| IBIS file stm32l0_71_72_73_81_82_83_lqfp48.ibs
| Created by s2ibis version 1.1 (customized version)
| North Carolina State University, ERL, 2006
[IBIS ver] 4.2
[File name] stm32l0_71_72_73_81_82_83_lqfp48.ibs
[File Rev] 1.0
[Date]  14-03-2016
[Source] Data Created at STMicroelectronics
[Notes]  File originated from ELDO simulations.
[Disclaimer]  This information is for modeling purpose only and is
   not guaranted. The information is subject to change without
   notice.
[Copyright] Copyright 2016 STMicroelectronics Inc.
|   Component stm32l0_71_72_73_81_82_83_lqfp48
[Component] stm32l0_71_72_73_81_82_83_lqfp48
[Manufacturer] STMicroelectronics
[Package]
| variable   typ   min   max
R_pkg   0.0   0.0   0.0
L_pkg   0.0H   0.0H   0.0H
C_pkg   0.0F   0.0F   0.0F
[Pin]  signal_name   model_name   R_pin   L_pin   C_pin
1 VLCD POWER   0.053   3.42534E-09   90.4E-15
2 PC13 io8p_wsudq_ls_ft_v33   48.4E-3   2.9E-9   64.4E-15
3 PC14-OSC32_IN io8p_wsudq_ls_ft_v33   44.7E-3   2.5E-9   43.7E-15
4 PC15-OSC32_OUT io8p_sudq_ls_tc_esdft 41.9E-3   2.2E-9   28.1E-15
5 PH0-OSC_IN io8p_sudq_ls_tc_esdft   40.1E-3   2.0E-9   17.7E-15
6 PH1-OSC_OUT io8p_sudq_ls_tc_esdft   0.03913   1.89021E-09   12.5E-15
7 NRST ioreset_ft_v33   0.03913   1.89021E-09   12.5E-15
8 VSSA GND   40.1E-3   2.0E-9   17.8E-15
9 VDDA POWER   41.9E-3   2.2E-9   28.2E-15
10 PA0 io8p_wsudq_ls_ft_v33   44.7E-3   2.5E-9   43.8E-15
11 PA1 io8p_wsudq_lcd4_ls_ft  48.4E-3   2.9E-9   64.6E-15
12 PA2 io8p_wsudq_lcd4_ls_ft  0.053   3.42534E-09   90.4E-15
13 PA3 io8p_wsudq_lcd4_ls_ft  0.053   3.4E-9   90.4E-15
14 PA4 io8p_wsudq_i2cin_ls_ft 48.4E-3   2.9E-9   64.4E-15
15 PA5 io8p_wsudq_i2cin_ls_ft 44.7E-3   2.5E-9   43.7E-15
16 PA6 io8p_wsudq_lcd4_ls_ft  41.9E-3   2.2E-9   28.1E-15
17 PA7 io8p_wsudq_lcd4_ls_ft  40.1E-3   2.0E-9   17.7E-15
18 PB0 io8p_wsudq_lcd4_ls_ft  0.03913   1.9E-9   12.5E-15
19 PB1 io8p_wsudq_lcd4_ls_ft  0.03913   1.9E-9   12.5E-15
20 PB2 io8p_wsudq_lcd4_ls_ft  40.1E-3   2.0E-9   17.8E-15
21 PB10 io8p_sudq_lcd4_i2cin_ls_ft   41.9E-3   2.2E-9   28.2E-15
22 PB11 io8p_sudq_lcd4_i2cin_ls_ft   44.7E-3   2.5E-9   43.8E-15
23 VSS GND   48.4E-3   2.9E-9   64.6E-15
24 VDD POWER   0.053   3.4E-9   90.4E-15
25 PB12 io8p_wsudq_lcd4_ls_ft   0.053   3.4E-9   90.4E-15
26 PB13 io8p_sudq_lcd4_i2cin_ls_ft   48.4E-3   2.9E-9   64.4E-15
27 PB14 io8p_sudq_lcd4_i2cin_ls_ft   44.7E-3   2.5E-9   43.7E-15
28 PB15 io8p_wsudq_lcd4_ls_ft   41.9E-3   2.2E-9   28.1E-15
29 PA8 io8p_sudq_lcd4_i2cin_ls_ft   40.1E-3   2.0E-9   17.7E-15
30 PA9 io8p_sudq_lcd4_i2cin_ls_ft   0.03913   1.9E-9   12.5E-15
31 PA10 io8p_sudq_lcd4_i2cin_ls_ft   0.03913   1.9E-9   12.5E-15
32 PA11 io8usb_ls_ft   40.1E-3   2.0E-9   17.8E-15
33 PA12 io8usb_ls_ft   41.9E-3   2.2E-9   28.2E-15
34 PA13 io8p_sudq_ls_ft   44.7E-3   2.5E-9   43.8E-15
35 VSS GND   48.4E-3   2.9E-9   64.6E-15
36 VDD_USB POWER   0.053   3.4E-9   90.4E-15
37 PA14 io8p_sudq_ls_ft   0.053   3.4E-9   90.4E-15
38 PA15 io8p_wsudq_lcd4_ls_ft   48.4E-3   2.9E-9   64.4E-15
39 PB3 io8p_wsudq_lcd4_ls_ft   44.7E-3   2.5E-9   43.7E-15
40 PB4 io8p_sudq_lcd4_i2cin_ls_ft 41.9E-3   2.2E-9   28.1E-15
41 PB5 io8p_wsudq_lcd4_ls_ft   40.1E-3   2.0E-9   17.7E-15
42 PB6 io8p_wsudq_i2cin_ls_ft   0.03913   1.9E-9   12.5E-15
43 PB7 io8p_wsudq_i2cin_ls_ft   0.03913   1.9E-9   12.5E-15
44 BOOT0 vpp_test_hv  40.1E-3   2.0E-9   17.8E-15
45 PB8 io8p_sudq_lcd4_i2cin_ls_ft   41.9E-3   2.2E-9   28.2E-15
46 PB9 io8p_sudq_lcd4_i2cin_ls_ft   44.7E-3   2.5E-9   43.8E-15
47 VSS GND   48.4E-3  2.9E-9   64.6E-15
48 VDD POWER   0.053   3.4E-9   90.4E-15
[Model Selector] io8p_sudq_ls_ft
io8p00_sudq_ls_ft_pd_lv  "SPEED00 1P8V, PD=40kOhm"
io8p00_sudq_ls_ft_pu_lv  "SPEED00 1P8V, PU=40kOhm"
io8p00_sudq_ls_ft_lv  "SPEED00 1P8V"
io8p01_sudq_ls_ft_pd_lv  "SPEED01 1P8V, PD=40kOhm"
io8p01_sudq_ls_ft_pu_lv  "SPEED01 1P8V, PU=40kOhm"
io8p01_sudq_ls_ft_lv  "SPEED01 1P8V"
io8p10_sudq_ls_ft_pd_lv  "SPEED10 1P8V, PD=40kOhm"
io8p10_sudq_ls_ft_pu_lv  "SPEED10 1P8V, PU=40kOhm"
io8p10_sudq_ls_ft_lv  "SPEED10 1P8V"
io8p11_sudq_ls_ft_pd_lv  "SPEED11 1P8V, PD=40kOhm"
io8p11_sudq_ls_ft_pu_lv  "SPEED11 1P8V, PU=40kOhm"
io8p11_sudq_ls_ft_lv  "SPEED11 1P8V"
io8p00_sudq_ls_ft_pd  "SPEED00, PD=40kOhm"
io8p00_sudq_ls_ft_pu  "SPEED00, PU=40kOhm"
io8p00_sudq_ls_ft  "SPEED00"
io8p01_sudq_ls_ft_pd  "SPEED01, PD=40kOhm"
io8p01_sudq_ls_ft_pu  "SPEED01, PU=40kOhm"
io8p01_sudq_ls_ft  "SPEED01"
io8p10_sudq_ls_ft_pd  "SPEED10, PD=40kOhm"
io8p10_sudq_ls_ft_pu  "SPEED10, PU=40kOhm"
io8p10_sudq_ls_ft  "SPEED10"
io8p11_sudq_ls_ft_pd  "SPEED11, PD=40kOhm"
io8p11_sudq_ls_ft_pu  "SPEED11, PU=40kOhm"
io8p11_sudq_ls_ft  "SPEED11"
[Model Selector] io8p_sudq_ls_tc_esdft
io8p00_sudq_ls_tc_esdft_pd_lv  "SPEED00 1P8V, PD=40kOhm"
io8p00_sudq_ls_tc_esdft_pu_lv  "SPEED00 1P8V, PU=40kOhm"
io8p00_sudq_ls_tc_esdft_lv  "SPEED00 1P8V"
io8p01_sudq_ls_tc_esdft_pd_lv  "SPEED01 1P8V, PD=40kOhm"
io8p01_sudq_ls_tc_esdft_pu_lv  "SPEED01 1P8V, PU=40kOhm"
io8p01_sudq_ls_tc_esdft_lv  "SPEED01 1P8V"
io8p10_sudq_ls_tc_esdft_pd_lv  "SPEED10 1P8V, PD=40kOhm"
io8p10_sudq_ls_tc_esdft_pu_lv  "SPEED10 1P8V, PU=40kOhm"
io8p10_sudq_ls_tc_esdft_lv  "SPEED10 1P8V"
io8p11_sudq_ls_tc_esdft_pd_lv  "SPEED11 1P8V, PD=40kOhm"
io8p11_sudq_ls_tc_esdft_pu_lv  "SPEED11 1P8V, PU=40kOhm"
io8p11_sudq_ls_tc_esdft_lv  "SPEED11 1P8V"
io8p00_sudq_ls_tc_esdft_pd  "SPEED00, PD=40kOhm"
io8p00_sudq_ls_tc_esdft_pu  "SPEED00, PU=40kOhm"
io8p00_sudq_ls_tc_esdft  "SPEED00"
io8p01_sudq_ls_tc_esdft_pd  "SPEED01, PD=40kOhm"
io8p01_sudq_ls_tc_esdft_pu  "SPEED01, PU=40kOhm"
io8p01_sudq_ls_tc_esdft  "SPEED01"
io8p10_sudq_ls_tc_esdft_pd  "SPEED10, PD=40kOhm"
io8p10_sudq_ls_tc_esdft_pu  "SPEED10, PU=40kOhm"
io8p10_sudq_ls_tc_esdft  "SPEED10"
io8p11_sudq_ls_tc_esdft_pd  "SPEED11, PD=40kOhm"
io8p11_sudq_ls_tc_esdft_pu  "SPEED11, PU=40kOhm"
io8p11_sudq_ls_tc_esdft  "SPEED11"
[Model Selector] io8p_wsudq_i2cin_ls_ft
io8p00_wsudq_i2cin_ls_ft_pd_lv  "SPEED00 1P8V, PD=40kOhm"
io8p00_wsudq_i2cin_ls_ft_pu_lv  "SPEED00 1P8V, PU=40kOhm"
io8p00_wsudq_i2cin_ls_ft_lv  "SPEED00 1P8V"
io8p01_wsudq_i2cin_ls_ft_pd_lv  "SPEED01 1P8V, PD=40kOhm"
io8p01_wsudq_i2cin_ls_ft_pu_lv  "SPEED01 1P8V, PU=40kOhm"
io8p01_wsudq_i2cin_ls_ft_lv  "SPEED01 1P8V"
io8p10_wsudq_i2cin_ls_ft_pd_lv  "SPEED10 1P8V, PD=40kOhm"
io8p10_wsudq_i2cin_ls_ft_pu_lv  "SPEED10 1P8V, PU=40kOhm"
io8p10_wsudq_i2cin_ls_ft_lv  "SPEED10 1P8V"
io8p11_wsudq_i2cin_ls_ft_pd_lv  "SPEED11 1P8V, PD=40kOhm"
io8p11_wsudq_i2cin_ls_ft_pu_lv  "SPEED11 1P8V, PU=40kOhm"
io8p11_wsudq_i2cin_ls_ft_lv  "SPEED11 1P8V"
io8p00_wsudq_i2cin_ls_ft_pd  "SPEED00, PD=40kOhm"
io8p00_wsudq_i2cin_ls_ft_pu  "SPEED00, PU=40kOhm"
io8p00_wsudq_i2cin_ls_ft  "SPEED00"
io8p01_wsudq_i2cin_ls_ft_pd  "SPEED01, PD=40kOhm"
io8p01_wsudq_i2cin_ls_ft_pu  "SPEED01, PU=40kOhm"
io8p01_wsudq_i2cin_ls_ft  "SPEED01"
io8p10_wsudq_i2cin_ls_ft_pd  "SPEED10, PD=40kOhm"
io8p10_wsudq_i2cin_ls_ft_pu  "SPEED10, PU=40kOhm"
io8p10_wsudq_i2cin_ls_ft  "SPEED10"
io8p11_wsudq_i2cin_ls_ft_pd  "SPEED11, PD=40kOhm"
io8p11_wsudq_i2cin_ls_ft_pu  "SPEED11, PU=40kOhm"
io8p11_wsudq_i2cin_ls_ft  "SPEED11"
[Model Selector] io8p_wsudq_lcd4_ls_ft
io8p00_wsudq_lcd4_ls_ft_pd_lv  "SPEED00 1P8V, PD=40kOhm"
io8p00_wsudq_lcd4_ls_ft_pu_lv  "SPEED00 1P8V, PU=40kOhm"
io8p00_wsudq_lcd4_ls_ft_lv  "SPEED00 1P8V"
io8p01_wsudq_lcd4_ls_ft_pd_lv  "SPEED01 1P8V, PD=40kOhm"
io8p01_wsudq_lcd4_ls_ft_pu_lv  "SPEED01 1P8V, PU=40kOhm"
io8p01_wsudq_lcd4_ls_ft_lv  "SPEED01 1P8V"
io8p10_wsudq_lcd4_ls_ft_pd_lv  "SPEED10 1P8V, PD=40kOhm"
io8p10_wsudq_lcd4_ls_ft_pu_lv  "SPEED10 1P8V, PU=40kOhm"
io8p10_wsudq_lcd4_ls_ft_lv  "SPEED10 1P8V"
io8p11_wsudq_lcd4_ls_ft_pd_lv  "SPEED11 1P8V, PD=40kOhm"
io8p11_wsudq_lcd4_ls_ft_pu_lv  "SPEED11 1P8V, PU=40kOhm"
io8p11_wsudq_lcd4_ls_ft_lv  "SPEED11 1P8V"
io8p00_wsudq_lcd4_ls_ft_pd  "SPEED00, PD=40kOhm"
io8p00_wsudq_lcd4_ls_ft_pu  "SPEED00, PU=40kOhm"
io8p00_wsudq_lcd4_ls_ft  "SPEED00"
io8p01_wsudq_lcd4_ls_ft_pd  "SPEED01, PD=40kOhm"
io8p01_wsudq_lcd4_ls_ft_pu  "SPEED01, PU=40kOhm"
io8p01_wsudq_lcd4_ls_ft  "SPEED01"
io8p10_wsudq_lcd4_ls_ft_pd  "SPEED10, PD=40kOhm"
io8p10_wsudq_lcd4_ls_ft_pu  "SPEED10, PU=40kOhm"
io8p10_wsudq_lcd4_ls_ft  "SPEED10"
io8p11_wsudq_lcd4_ls_ft_pd  "SPEED11, PD=40kOhm"
io8p11_wsudq_lcd4_ls_ft_pu  "SPEED11, PU=40kOhm"
io8p11_wsudq_lcd4_ls_ft  "SPEED11"
[Model Selector] io8p_wsudq_ls_ft_v33
io8p00_wsudq_ls_ft_v33_pd_lv  "SPEED00 1P8V, PD=40kOhm"
io8p00_wsudq_ls_ft_v33_pu_lv  "SPEED00 1P8V, PU=40kOhm"
io8p00_wsudq_ls_ft_v33_lv  "SPEED00 1P8V"
io8p01_wsudq_ls_ft_v33_pd_lv  "SPEED01 1P8V, PD=40kOhm"
io8p01_wsudq_ls_ft_v33_pu_lv  "SPEED01 1P8V, PU=40kOhm"
io8p01_wsudq_ls_ft_v33_lv  "SPEED01 1P8V"
io8p10_wsudq_ls_ft_v33_pd_lv  "SPEED10 1P8V, PD=40kOhm"
io8p10_wsudq_ls_ft_v33_pu_lv  "SPEED10 1P8V, PU=40kOhm"
io8p10_wsudq_ls_ft_v33_lv  "SPEED10 1P8V"
io8p11_wsudq_ls_ft_v33_pd_lv  "SPEED11 1P8V, PD=40kOhm"
io8p11_wsudq_ls_ft_v33_pu_lv  "SPEED11 1P8V, PU=40kOhm"
io8p11_wsudq_ls_ft_v33_lv  "SPEED11 1P8V"
io8p00_wsudq_ls_ft_v33_pd  "SPEED00, PD=40kOhm"
io8p00_wsudq_ls_ft_v33_pu  "SPEED00, PU=40kOhm"
io8p00_wsudq_ls_ft_v33  "SPEED00"
io8p01_wsudq_ls_ft_v33_pd  "SPEED01, PD=40kOhm"
io8p01_wsudq_ls_ft_v33_pu  "SPEED01, PU=40kOhm"
io8p01_wsudq_ls_ft_v33  "SPEED01"
io8p10_wsudq_ls_ft_v33_pd  "SPEED10, PD=40kOhm"
io8p10_wsudq_ls_ft_v33_pu  "SPEED10, PU=40kOhm"
io8p10_wsudq_ls_ft_v33  "SPEED10"
io8p11_wsudq_ls_ft_v33_pd  "SPEED11, PD=40kOhm"
io8p11_wsudq_ls_ft_v33_pu  "SPEED11, PU=40kOhm"
io8p11_wsudq_ls_ft_v33  "SPEED11"
[Model Selector] vpp_test_hv
vpp_test_hv_2p4  "Input Buffer 1P65V"
vpp_test_hv_3p3  "Input Buffer"
[Model Selector] io8usb_ls_ft
io8usb_ls_ft_dpdn_pu  "HS USB DP/DN IO + PU=1.2kOhm"
io8usb_ls_ft_dpdn  "HS USB DP/DN IO"
io8p00_ls_ft_pd_lv  "SPEED00 1P8V, PD=40kOhm"
io8p00_ls_ft_pu_lv  "SPEED00 1P8V, PU=40kOhm"
io8p00_ls_ft_lv  "SPEED00 1P8V"
io8p01_ls_ft_pd_lv  "SPEED01 1P8V, PD=40kOhm"
io8p01_ls_ft_pu_lv  "SPEED01 1P8V, PU=40kOhm"
io8p01_ls_ft_lv  "SPEED01 1P8V"
io8p10_ls_ft_pd_lv  "SPEED10 1P8V, PD=40kOhm"
io8p10_ls_ft_pu_lv  "SPEED10 1P8V, PU=40kOhm"
io8p10_ls_ft_lv  "SPEED10 1P8V"
io8p11_ls_ft_pd_lv  "SPEED11 1P8V, PD=40kOhm"
io8p11_ls_ft_pu_lv  "SPEED11 1P8V, PU=40kOhm"
io8p11_ls_ft_lv  "SPEED11 1P8V"
io8p00_ls_ft_pd  "SPEED00, PD=40kOhm"
io8p00_ls_ft_pu  "SPEED00, PU=40kOhm"
io8p00_ls_ft  "SPEED00"
io8p01_ls_ft_pd  "SPEED01, PD=40kOhm"
io8p01_ls_ft_pu  "SPEED01, PU=40kOhm"
io8p01_ls_ft  "SPEED01"
io8p10_ls_ft_pd  "SPEED10, PD=40kOhm"
io8p10_ls_ft_pu  "SPEED10, PU=40kOhm"
io8p10_ls_ft  "SPEED10"
io8p11_ls_ft_pd  "SPEED11, PD=40kOhm"
io8p11_ls_ft_pu  "SPEED11, PU=40kOhm"
io8p11_ls_ft  "SPEED11"
[Model Selector] io8p_sudq_lcd4_i2cin_ls_ft
io8p00_sudq_lcd4_i2cin_ls_ft_pd_lv  "SPEED00 1P8V, PD=40kOhm"
io8p00_sudq_lcd4_i2cin_ls_ft_pu_lv  "SPEED00 1P8V, PU=40kOhm"
io8p00_sudq_lcd4_i2cin_ls_ft_lv  "SPEED00 1P8V"
io8p01_sudq_lcd4_i2cin_ls_ft_pd_lv  "SPEED01 1P8V, PD=40kOhm"
io8p01_sudq_lcd4_i2cin_ls_ft_pu_lv  "SPEED01 1P8V, PU=40kOhm"
io8p01_sudq_lcd4_i2cin_ls_ft_lv  "SPEED01 1P8V"
io8p10_sudq_lcd4_i2cin_ls_ft_pd_lv  "SPEED10 1P8V, PD=40kOhm"
io8p10_sudq_lcd4_i2cin_ls_ft_pu_lv  "SPEED10 1P8V, PU=40kOhm"
io8p10_sudq_lcd4_i2cin_ls_ft_lv  "SPEED10 1P8V"
io8p11_sudq_lcd4_i2cin_ls_ft_pd_lv  "SPEED11 1P8V, PD=40kOhm"
io8p11_sudq_lcd4_i2cin_ls_ft_pu_lv  "SPEED11 1P8V, PU=40kOhm"
io8p11_sudq_lcd4_i2cin_ls_ft_lv  "SPEED11 1P8V"
io8p00_sudq_lcd4_i2cin_ls_ft_pd  "SPEED00, PD=40kOhm"
io8p00_sudq_lcd4_i2cin_ls_ft_pu  "SPEED00, PU=40kOhm"
io8p00_sudq_lcd4_i2cin_ls_ft  "SPEED00"
io8p01_sudq_lcd4_i2cin_ls_ft_pd  "SPEED01, PD=40kOhm"
io8p01_sudq_lcd4_i2cin_ls_ft_pu  "SPEED01, PU=40kOhm"
io8p01_sudq_lcd4_i2cin_ls_ft  "SPEED01"
io8p10_sudq_lcd4_i2cin_ls_ft_pd  "SPEED10, PD=40kOhm"
io8p10_sudq_lcd4_i2cin_ls_ft_pu  "SPEED10, PU=40kOhm"
io8p10_sudq_lcd4_i2cin_ls_ft  "SPEED10"
io8p11_sudq_lcd4_i2cin_ls_ft_pd  "SPEED11, PD=40kOhm"
io8p11_sudq_lcd4_i2cin_ls_ft_pu  "SPEED11, PU=40kOhm"
io8p11_sudq_lcd4_i2cin_ls_ft  "SPEED11"
[Model Selector] ioreset_ft_v33
ioreset_ft_v33_pu_lv  "ioreset 1P8V + PU=40kOhm"
ioreset_ft_v33_nopu_lv  "ioreset 1P8V"
ioreset_ft_v33_pu  "ioreset + PU=40kOhm"
ioreset_ft_v33_nopu  "ioreset"
| Models and submodels in the file (176): io8p00_sudq_ls_ft_pd_lv (I/O), io8p00_sudq_ls_ft_pu_lv (I/O), io8p00_sudq_ls_ft_lv (I/O), io8p01_sudq_ls_ft_pd_lv (I/O), io8p01_sudq_ls_ft_pu_lv (I/O), io8p01_sudq_ls_ft_lv (I/O), io8p10_sudq_ls_ft_pd_lv (I/O), io8p10_sudq_ls_ft_pu_lv (I/O), io8p10_sudq_ls_ft_lv (I/O), io8p11_sudq_ls_ft_pd_lv (I/O), io8p11_sudq_ls_ft_pu_lv (I/O), io8p11_sudq_ls_ft_lv (I/O), io8p00_sudq_ls_ft_pd (I/O), io8p00_sudq_ls_ft_pu (I/O), io8p00_sudq_ls_ft (I/O), io8p01_sudq_ls_ft_pd (I/O), io8p01_sudq_ls_ft_pu (I/O), io8p01_sudq_ls_ft (I/O), io8p10_sudq_ls_ft_pd (I/O), io8p10_sudq_ls_ft_pu (I/O), io8p10_sudq_ls_ft (I/O), io8p11_sudq_ls_ft_pd (I/O), io8p11_sudq_ls_ft_pu (I/O), io8p11_sudq_ls_ft (I/O), io8p00_sudq_ls_tc_esdft_pd_lv (I/O), io8p00_sudq_ls_tc_esdft_pu_lv (I/O), io8p00_sudq_ls_tc_esdft_lv (I/O), io8p01_sudq_ls_tc_esdft_pd_lv (I/O), io8p01_sudq_ls_tc_esdft_pu_lv (I/O), io8p01_sudq_ls_tc_esdft_lv (I/O), io8p10_sudq_ls_tc_esdft_pd_lv (I/O), io8p10_sudq_ls_tc_esdft_pu_lv (I/O), io8p10_sudq_ls_tc_esdft_lv (I/O), io8p11_sudq_ls_tc_esdft_pd_lv (I/O), io8p11_sudq_ls_tc_esdft_pu_lv (I/O), io8p11_sudq_ls_tc_esdft_lv (I/O), io8p00_sudq_ls_tc_esdft_pd (I/O), io8p00_sudq_ls_tc_esdft_pu (I/O), io8p00_sudq_ls_tc_esdft (I/O), io8p01_sudq_ls_tc_esdft_pd (I/O), io8p01_sudq_ls_tc_esdft_pu (I/O), io8p01_sudq_ls_tc_esdft (I/O), io8p10_sudq_ls_tc_esdft_pd (I/O), io8p10_sudq_ls_tc_esdft_pu (I/O), io8p10_sudq_ls_tc_esdft (I/O), io8p11_sudq_ls_tc_esdft_pd (I/O), io8p11_sudq_ls_tc_esdft_pu (I/O), io8p11_sudq_ls_tc_esdft (I/O), io8p00_wsudq_i2cin_ls_ft_pd_lv (I/O), io8p00_wsudq_i2cin_ls_ft_pu_lv (I/O), io8p00_wsudq_i2cin_ls_ft_lv (I/O), io8p01_wsudq_i2cin_ls_ft_pd_lv (I/O), io8p01_wsudq_i2cin_ls_ft_pu_lv (I/O), io8p01_wsudq_i2cin_ls_ft_lv (I/O), io8p10_wsudq_i2cin_ls_ft_pd_lv (I/O), io8p10_wsudq_i2cin_ls_ft_pu_lv (I/O), io8p10_wsudq_i2cin_ls_ft_lv (I/O), io8p11_wsudq_i2cin_ls_ft_pd_lv (I/O), io8p11_wsudq_i2cin_ls_ft_pu_lv (I/O), io8p11_wsudq_i2cin_ls_ft_lv (I/O), io8p00_wsudq_i2cin_ls_ft_pd (I/O), io8p00_wsudq_i2cin_ls_ft_pu (I/O), io8p00_wsudq_i2cin_ls_ft (I/O), io8p01_wsudq_i2cin_ls_ft_pd (I/O), io8p01_wsudq_i2cin_ls_ft_pu (I/O), io8p01_wsudq_i2cin_ls_ft (I/O), io8p10_wsudq_i2cin_ls_ft_pd (I/O), io8p10_wsudq_i2cin_ls_ft_pu (I/O), io8p10_wsudq_i2cin_ls_ft (I/O), io8p11_wsudq_i2cin_ls_ft_pd (I/O), io8p11_wsudq_i2cin_ls_ft_pu (I/O), io8p11_wsudq_i2cin_ls_ft (I/O), io8p00_wsudq_lcd4_ls_ft_pd_lv (I/O), io8p00_wsudq_lcd4_ls_ft_pu_lv (I/O), io8p00_wsudq_lcd4_ls_ft_lv (I/O), io8p01_wsudq_lcd4_ls_ft_pd_lv (I/O), io8p01_wsudq_lcd4_ls_ft_pu_lv (I/O), io8p01_wsudq_lcd4_ls_ft_lv (I/O), io8p10_wsudq_lcd4_ls_ft_pd_lv (I/O), io8p10_wsudq_lcd4_ls_ft_pu_lv (I/O)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
